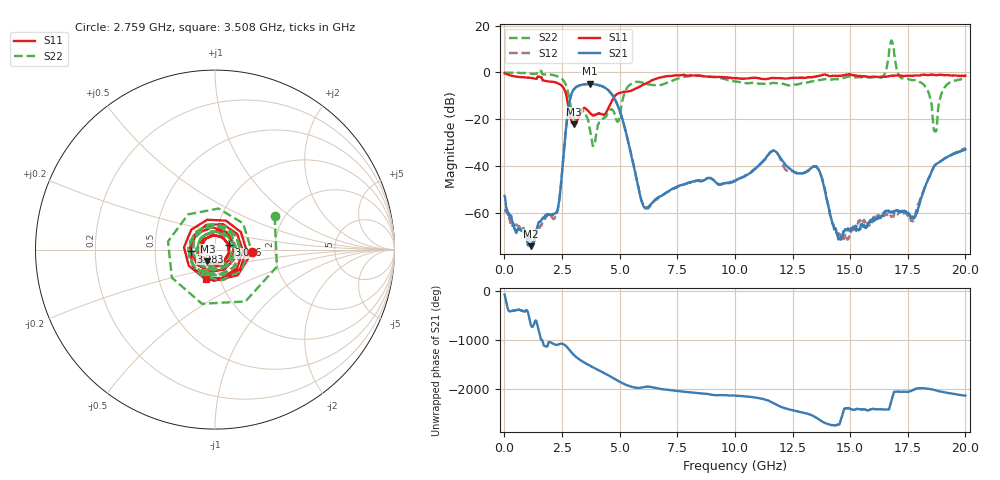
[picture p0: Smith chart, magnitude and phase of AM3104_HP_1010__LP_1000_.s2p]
!Created with skrf (http://scikit-rf.org).
# Hz S RI R 50.0
!freq ReS11 ImS11 ReS21 ImS21 ReS12 ImS12 ReS22 ImS22
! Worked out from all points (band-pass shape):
!   1601 points, 10 MHz to 20 GHz, reference 50 ohm
!   highest |S21| = -4.84 dB at 3.708 GHz (marker M1); lowest = -74.1 dB at 1.134 GHz (marker M2)
!   |S21| within 3 dB of the highest: 2.97 GHz to 4.541 GHz (1.571 GHz wide, 41.8 % of centre)
!   lowest |S11| = -22.2 dB at 3.021 GHz (marker M3), VSWR 1.17, Z = 45.5 - j5.98 ohm
!   |S11| at or under -10 dB: 2.691 GHz to 4.794 GHz (2.104 GHz wide, 56.2 % of centre)
!   |S22| runs from -31.4 to 13.7 dB; largest |S21 - S12| = 0.043
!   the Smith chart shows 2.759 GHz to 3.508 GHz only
!   S11 on the Smith chart (normalised r, x): 2.759 GHz: 1.52, -0.04; 3.096 GHz: 1.17, +0.06; 3.283 GHz: 0.76, -0.02; 3.508 GHz: 0.86, -0.29
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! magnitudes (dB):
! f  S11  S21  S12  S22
! 10 MHz  -0.4  -52.7  -59.3  0.0
! 1.134 GHz  -2.3  -74.1  -71.3  -0.5
! 2.271 GHz  -4.4  -59.3  -60.5  -1.6
! 2.759 GHz  -13.7  -16.7  -16.7  -8.4
! 3.021 GHz  -22.2  -7.1  -7.1  -19.3
! 3.096 GHz  -21.8  -6.3  -6.3  -20.4
! 3.283 GHz  -17.3  -5.4  -5.5  -18.1
! 3.346 GHz  -16.1  -5.3  -5.4  -16.9
! 3.508 GHz  -15.3  -5.0  -5.1  -17.2
! 3.708 GHz  -17.1  -4.8  -4.9  -24.2
! 4.87 GHz  -9.3  -13.0  -13.0  -20.5
! 6.044 GHz  -5.1  -57.2  -56.9  -4.5
! 6.682 GHz  -2.3  -53.2  -53.5  -5.4
! 10.01 GHz  -2.5  -46.3  -46.5  -3.9
! 11.64 GHz  -2.4  -33.5  -33.4  -4.4
! 13.34 GHz  -2.1  -40.6  -40.6  -3.9
! 14.53 GHz  -1.4  -70.6  -69.1  -2.9
! 16.68 GHz  -1.6  -59.3  -61.3  7.3
! 17.81 GHz  -1.3  -61.4  -61.2  -3.3
! 18.69 GHz  -1.1  -39.5  -39.5  -25.2
! 19.09 GHz  -1.2  -36.7  -36.8  -6.5
! 20 GHz  -1.4  -32.8  -32.3  -2.6
